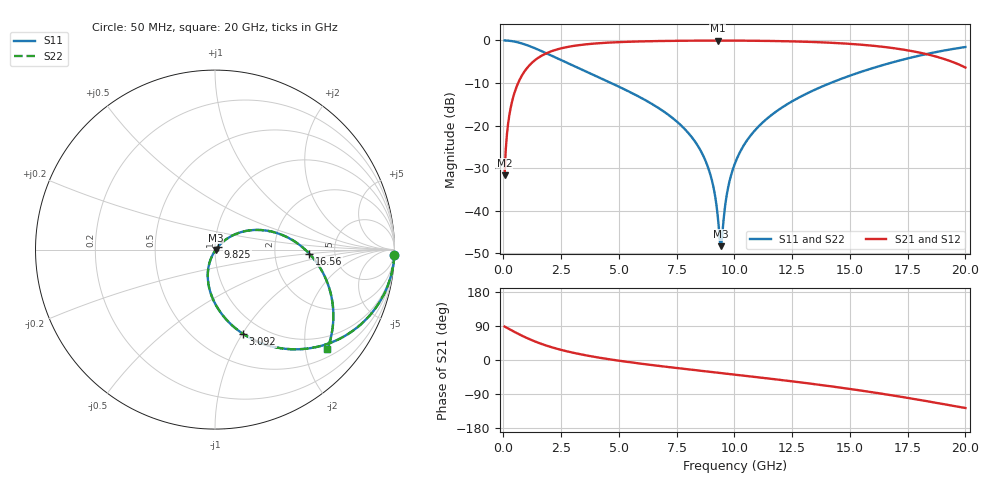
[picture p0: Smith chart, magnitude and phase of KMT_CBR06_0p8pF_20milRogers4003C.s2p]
! Data measured by Modelithics Inc. support@modelithics.com 813-866-6335
! KEMET CBR0603 0.8pF, Pad Width= 0.851mm, Pad Length= 0.64mm, Pad Gap= 0.62mm, 20mil Rogers 4003C substrate Data, January 2022
# hz S ma R 50
! 2 Port Network Data from SP1.SP block
! freq  magS11  angS11  magS21  angS21  magS12  angS12  magS22  angS22
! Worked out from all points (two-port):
!   401 points, 50 MHz to 20 GHz, reference 50 ohm
!   highest |S21| = -0.04 dB at 9.277 GHz (marker M1); lowest = -31.6 dB at 50 MHz (marker M2)
!   |S21| within 3 dB of the highest: 1.853 GHz to 18.17 GHz (16.32 GHz wide, 163 % of centre)
!   lowest |S11| = -48.3 dB at 9.427 GHz (marker M3), VSWR 1.01, Z = 50.4 - j0.147 ohm
!   |S11| at or under -10 dB: 4.658 GHz to 14.16 GHz (9.503 GHz wide, 101 % of centre)
!   |S22| runs from -48.3 to 0.0 dB; largest |S21 - S12| = 0
!   S11 on the Smith chart (normalised r, x): 50 MHz: 1, -68; 3.092 GHz: 0.81, -1.01; 9.825 GHz: 1.04, +0.03; 16.56 GHz: 3.20, -0.20; 20 GHz: 0.67, -2.48
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5e7  0.9997 -1.7  0.02616 88.3  0.02616 88.3  0.9997 -1.7
1.99625e8  0.9946 -6.7  0.1039 83.3  0.1039 83.3  0.9946 -6.7
3.4925e8  0.9836 -11.7  0.1799 78.3  0.1799 78.3  0.9836 -11.7
8.48e8  0.9129 -27.2  0.4074 62.8  0.4074 62.8  0.9129 -27.2
1.695875e9  0.7397 -48.5  0.6716 41.4  0.6716 41.4  0.7397 -48.5
3.092375e9  0.4944 -71.6  0.8672 18.2  0.8672 18.2  0.4944 -71.6
3.391625e9  0.4538 -75.3  0.8889 14.4  0.8889 14.4  0.4538 -75.3
6.73325e9  0.1595 -104.6  0.9841 -15.6  0.9841 -15.6  0.1595 -104.6
7.780625e9  0.095 -111.2  0.9921 -23.1  0.9921 -23.1  0.095 -111.2
8.52875e9  0.05125 -114.5  0.995 -28.3  0.995 -28.3  0.05125 -114.5
9.0275e9  0.02258 -112.6  0.9959 -31.7  0.9959 -31.7  0.02258 -112.6
9.276875e9  0.008688 -98.4  0.996 -33.5  0.996 -33.5  0.008688 -98.4
9.4265e9  0.003828 -22.4  0.9959 -34.5  0.9959 -34.5  0.003828 -22.4
9.8255e9  0.02439 43.5  0.9954 -37.2  0.9954 -37.2  0.02439 43.5
1.0025e10  0.03603 45.0  0.995 -38.6  0.995 -38.6  0.03603 45.0
1.047388e10  0.0627 44.4  0.9934 -41.7  0.9934 -41.7  0.0627 44.4
1.117212e10  0.1055 40.8  0.9893 -46.6  0.9893 -46.6  0.1055 40.8
1.336662e10  0.255 25.5  0.9594 -62.9  0.9594 -62.9  0.255 25.5
1.655862e10  0.5258 -2.5  0.8335 -90.7  0.8335 -90.7  0.5258 -2.5
1.670825e10  0.5398 -3.9  0.8239 -92.1  0.8239 -92.1  0.5398 -3.9
1.855362e10  0.7141 -23.8  0.6657 -111.0  0.6657 -111.0  0.7141 -23.8
2e10  0.8365 -41.5  0.4804 -126.7  0.4804 -126.7  0.8365 -41.5
